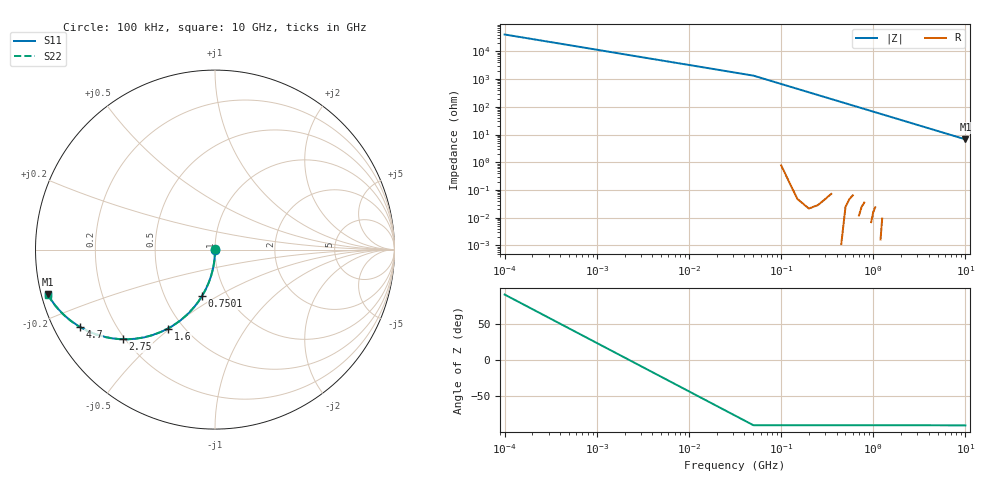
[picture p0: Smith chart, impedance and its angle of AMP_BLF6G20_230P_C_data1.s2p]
! Created Tue Aug  7 13:29:10 2007
# hz S ri R 50
! 2 Port Network Data from SP1.SP block
! freq  reS11  imS11  reS21  imS21  reS12  imS12  reS22  imS22
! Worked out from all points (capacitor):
!   201 points, 100 kHz to 10 GHz, reference 50 ohm
!   read as one part in shunt: C = 2.37 pF near 50.1 MHz
!   lowest |Z| = 6.76 ohm at 10 GHz (marker M1)
!   S11 on the Smith chart (normalised r, x): 100 kHz: 1.00, +0.00; 750.1 MHz: 0.76, -0.43; 1.6 GHz: 0.41, -0.49; 2.75 GHz: 0.19, -0.39; 4.7 GHz: 0.08, -0.26; 10 GHz: 0.02, -0.13
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100000  1.62e-05 0.000526  1 0.000606  1 0.000606  1.61e-05 0.000699
5.01e7  -0.000313 -0.0184  0.9996 -0.0187  0.9996 -0.0187  -0.000312 -0.0187
1.001e8  -0.00139 -0.0366  0.9985 -0.0373  0.9985 -0.0373  -0.00139 -0.0372
1.501e8  -0.00312 -0.0564  0.9968 -0.056  0.9968 -0.056  -0.00312 -0.0559
2.001e8  -0.00552 -0.0745  0.9944 -0.0744  0.9944 -0.0744  -0.00552 -0.0742
2.501e8  -0.00859 -0.0923  0.9913 -0.0926  0.9913 -0.0926  -0.00858 -0.0923
3.501e8  -0.0168 -0.1277  0.9831 -0.1287  0.9831 -0.1287  -0.0167 -0.1284
5.001e8  -0.0336 -0.18  0.9662 -0.1805  0.9662 -0.1805  -0.0336 -0.1801
6.501e8  -0.0555 -0.2292  0.9443 -0.2293  0.9443 -0.2293  -0.0555 -0.2288
7.501e8  -0.0726 -0.259  0.9272 -0.2597  0.9272 -0.2597  -0.0725 -0.2591
1.1001e9  -0.1441 -0.3513  0.8557 -0.3516  0.8557 -0.3516  -0.1439 -0.3508
1.6001e9  -0.2625 -0.4396  0.7371 -0.4407  0.7371 -0.4407  -0.2623 -0.4397
1.7001e9  -0.2867 -0.4511  0.713 -0.4529  0.713 -0.4529  -0.2864 -0.4519
2.1501e9  -0.3912 -0.4882  0.6083 -0.4888  0.6083 -0.4888  -0.3908 -0.4878
2.7501e9  -0.5126 -0.4988  0.4869 -0.5008  0.4869 -0.5008  -0.512 -0.4997
3.3501e9  -0.6095 -0.4873  0.39 -0.489  0.39 -0.489  -0.6088 -0.4879
4.0001e9  -0.69 -0.4622  0.3095 -0.4639  0.3095 -0.4639  -0.6892 -0.4627
4.7001e9  -0.7545 -0.4287  0.2449 -0.4319  0.2449 -0.4319  -0.7537 -0.4307
5.0001e9  -0.7767 -0.4145  0.2227 -0.4181  0.2227 -0.4181  -0.7759 -0.4169
6.7001e9  -0.862 -0.3427  0.1372 -0.3469  0.1372 -0.3469  -0.8612 -0.3456
8.3501e9  -0.9065 -0.2891  0.0924 -0.2934  0.0924 -0.2934  -0.9058 -0.2919
1.00001e10  -0.9329 -0.2469  0.0659 -0.2527  0.0659 -0.2527  -0.9323 -0.251
